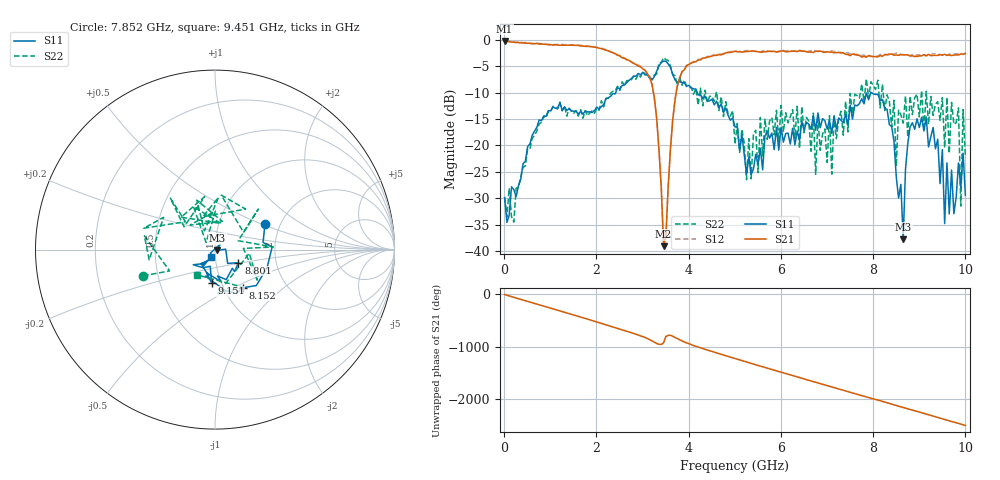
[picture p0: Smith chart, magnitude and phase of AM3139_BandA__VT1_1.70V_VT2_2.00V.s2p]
! Date/Time: Tue, Nov 13, 2018 4:57 PM
! Network Analyzer: Agilent Technologies E8364B Rev: A.07.50.67
! Sweep from 0.010 to 10.000 GHz, 201 Points, Sweep Type: LIN
! Power Supply: 1.701 V, 0.000 A
# Hz S DB R 50
!freq MagS11 AngS11 MagS21 AngS21 MagS12 AngS12 MagS22 AngS22
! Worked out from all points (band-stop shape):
!   201 points, 10 MHz to 10 GHz, reference 50 ohm
!   highest |S21| = -0.23 dB at 10 MHz (marker M1); lowest = -39.1 dB at 3.457 GHz (marker M2)
!   |S21| within 3 dB of the highest: start of sweep to 2.531 GHz; 4.437 GHz to 7.744 GHz (3.307 GHz wide, 54.3 % of centre)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
!   lowest |S11| = -37.8 dB at 8.651 GHz (marker M3), VSWR 1.03, Z = 51.3 - j0.383 ohm
!   |S11| at or under -10 dB: start of sweep to 2.418 GHz; 4.185 GHz to 7.95 GHz (3.764 GHz wide, 62 % of centre); 7.963 GHz to end of sweep
!   |S22| runs from -34.5 to -3.4 dB; largest |S21 - S12| = 0.033
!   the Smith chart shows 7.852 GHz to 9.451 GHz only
!   S11 on the Smith chart (normalised r, x): 7.852 GHz: 1.67, +0.53; 8.152 GHz: 1.23, -0.56; 8.801 GHz: 1.29, -0.19; 9.151 GHz: 0.90, -0.34; 9.451 GHz: 0.96, -0.07
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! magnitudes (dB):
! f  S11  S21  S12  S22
! 10 MHz  -29.9  -0.2  -0.1  -29.8
! 1.708 GHz  -14.1  -1.2  -1.1  -14.9
! 3.057 GHz  -6.5  -5.8  -5.8  -6.7
! 3.357 GHz  -5.0  -20.9  -20.8  -4.4
! 3.457 GHz  -4.0  -39.1  -38.7  -3.4
! 3.806 GHz  -7.9  -7.2  -7.2  -7.1
! 5.005 GHz  -16.5  -2.2  -2.2  -19.8
! 6.703 GHz  -14.4  -2.4  -2.2  -13.9
! 6.753 GHz  -17.1  -2.2  -2.1  -25.5
! 7.103 GHz  -17.7  -2.4  -2.1  -25.4
! 7.852 GHz  -10.1  -3.3  -3.2  -7.4
! 8.152 GHz  -11.6  -3.0  -2.8  -12.9
! 8.352 GHz  -16.1  -2.7  -2.8  -11.7
! 8.501 GHz  -26.0  -2.9  -2.5  -24.0
! 8.651 GHz  -37.8  -2.8  -2.8  -15.8
! 8.801 GHz  -16.5  -3.1  -3.0  -10.7
! 9.151 GHz  -14.6  -3.0  -3.1  -9.8
! 9.451 GHz  -27.2  -2.8  -2.8  -15.3
! 9.85 GHz  -23.3  -2.9  -2.7  -12.9
! 9.9 GHz  -28.0  -2.7  -2.7  -31.5
! 9.95 GHz  -21.5  -2.7  -2.8  -13.2
! 10 GHz  -29.5  -2.6  -2.5  -22.3
